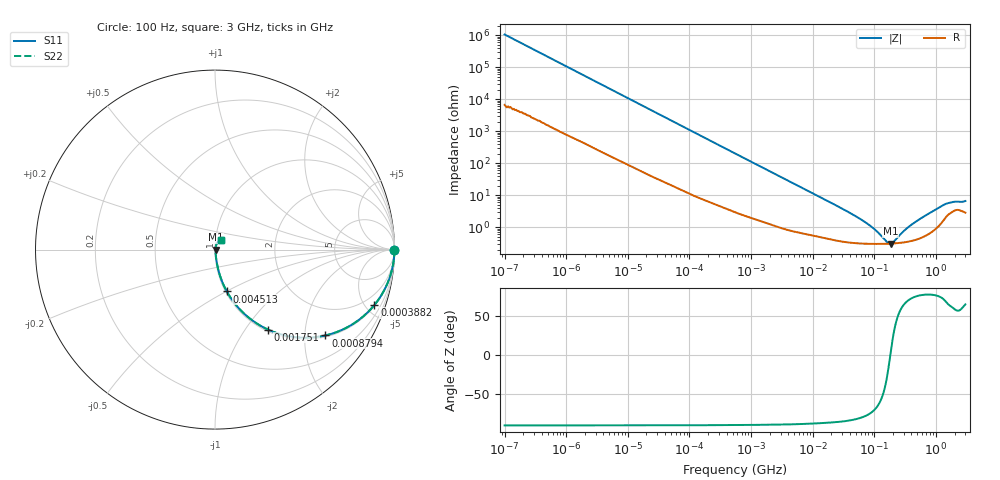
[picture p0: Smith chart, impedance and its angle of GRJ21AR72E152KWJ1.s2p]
!Murata Part Number: GRJ21AR72E152KWJ1
!These Parameters are Measured in Series Mode Connection
!Data Generated on Jun 19, 2026
!  o--ll--o
!Port1  Port2
!  o------o
!Operation Temp=25[degC], DC Bias Voltage=0[V]
!Freq. Start=100[Hz] Stop=3[GHz] 401[Steps]
# Hz S RI R 50
!Freq.(Hz) S11(Real) S11(Imag) S21(Real) S21(Imag) S12(Real) S12(Imag) S22(Real) S22(Imag)
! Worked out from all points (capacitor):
!   401 points, 100 Hz to 3 GHz, reference 50 ohm
!   read as one part in series: C = 1.5 nF near 109 Hz
!   lowest |Z| = 308 mohm at 182.8 MHz (marker M1)
!   series resonance near 181.6 MHz, so ESL is about 510 pH
!   S11 on the Smith chart (normalised r, x): 100 Hz: open; 388.2 kHz: 1.08, -5.72; 879.4 kHz: 1.04, -2.54; 1.751 MHz: 1.03, -1.28; 4.513 MHz: 1.02, -0.50; 3 GHz: 1.06, +0.12
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100  1 -9.41e-05  6e-07 9.41e-05  6e-07 9.41e-05  1 -9.41e-05
1788  1 -0.00166  1.55e-05 0.00166  1.55e-05 0.00166  1 -0.00166
31977  0.9989 -0.0292  0.00112 0.0292  0.00112 0.0292  0.9989 -0.0292
132342  0.9846 -0.1181  0.0154 0.1181  0.0154 0.1181  0.9846 -0.1181
388167  0.8878 -0.309  0.1122 0.309  0.1122 0.309  0.8878 -0.309
547723  0.8016 -0.3916  0.1984 0.3916  0.1984 0.3916  0.8016 -0.3916
879390  0.6156 -0.4782  0.3844 0.4782  0.3844 0.4782  0.6156 -0.4782
1750920  0.2962 -0.4461  0.7038 0.4461  0.7038 0.4461  0.2962 -0.4461
2692740  0.1558 -0.3507  0.8442 0.3507  0.8442 0.3507  0.1558 -0.3507
4513443  0.0659 -0.2333  0.9341 0.2333  0.9341 0.2333  0.0659 -0.2333
9794414  0.0188 -0.1142  0.9812 0.1142  0.9812 0.1142  0.0188 -0.1142
6.508213e7  0.00331 -0.0157  0.9967 0.0157  0.9967 0.0157  0.00331 -0.0157
1.000898e8  0.00307 -0.00817  0.9969 0.00817  0.9969 0.00817  0.00307 -0.00817
1.539281e8  0.00304 -0.00215  0.997 0.00215  0.997 0.00215  0.00304 -0.00215
1.751444e8  0.00306 -0.000468  0.9969 0.000468  0.9969 0.000468  0.00306 -0.000468
1.828475e8  0.00307 8.89e-05  0.9969 -8.89e-05  0.9969 -8.89e-05  0.00307 8.89e-05
2.080499e8  0.00312 0.00177  0.9969 -0.00177  0.9969 -0.00177  0.00312 0.00177
2.935688e8  0.00337 0.00646  0.9966 -0.00646  0.9966 -0.00646  0.00337 0.00646
4.142403e8  0.00391 0.0119  0.9961 -0.0119  0.9961 -0.0119  0.00391 0.0119
1.214989e9  0.0149 0.042  0.9851 -0.042  0.9851 -0.042  0.0149 0.042
1.789813e9  0.0309 0.0498  0.9691 -0.0498  0.9691 -0.0498  0.0309 0.0498
3e9  0.0311 0.056  0.9689 -0.056  0.9689 -0.056  0.0311 0.056
